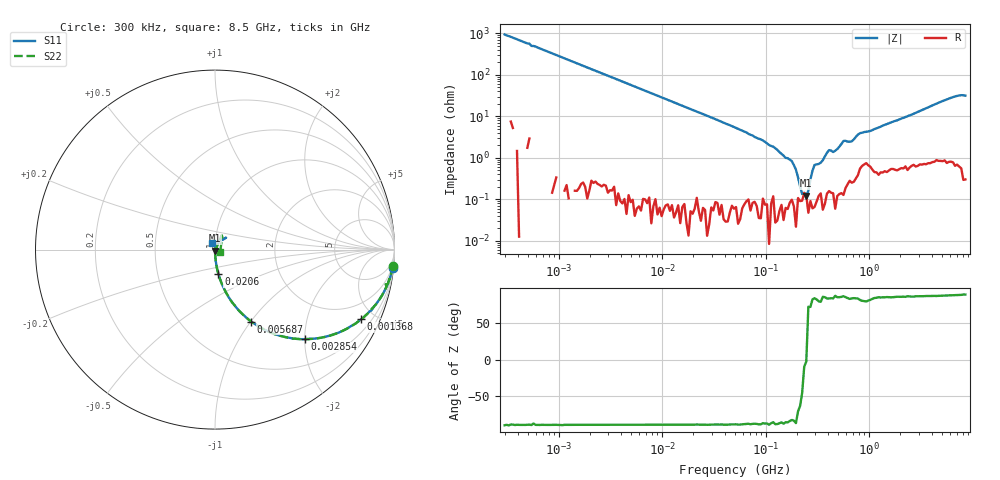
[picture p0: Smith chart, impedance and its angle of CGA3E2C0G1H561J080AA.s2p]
! S-parameter Generated by TDK Corporation
! Copyright(C) 2015 TDK Corporation.
! All Rights Reserved.
! TDK P/N: CGA3E2C0G1H561J080AA (Multilayer Ceramic Chip Capacitors)
! Property: C=560pF
! Size(LxWxT): 1.6x0.8x0.8mm, 0.063x0.031x0.031inches
! Model Type: s2p (Touchstone File Format Version 1.0)
! Frequency: DC=Yes Start=0.3MHz Stop=8500MHz 225points Log-sweep
! Note:
! Model Generated on Jun. 23, 2015
! Hash(MD5):
! Port Assignments:
!  1 ---| |--- 2
! Applicable Conditions:
!  Temperature = 25 degC
!  DC Bias Voltage = 0 V
!  Small Signal Operation
! Terms and conditions regarding TDK Simulation Models
! (1)This simulation model is being provided solely for informational purposes. Please refer to the specifications of the products in terms of detailed characteristics of such products.
! (2)In no event shall TDK Corporation of any of its subsidiaries be liable for any loss or damage arising, directly or indirectly,
!  From any information contained in this simulation model, including, but not limited to loss or damages arising from any inaccuracies, omissions or errors in connection with such information.
! (3)Any and all copyrights on this simulation model are owned by TDK Corporation.
!  Duplication or redistribution of this simulation model without prior written permission from TDK Corporation is prohibited.
! (4)This simulation model is subject to any modification or change without any prior notice.
! (5)Neither TDK Corporation nor any of its subsidiaries shall make any warranty, express or implied,
!  Including but not limited to the correctness, implied warranties of merchantability and fitness for a particular purpose with respect to this simulation models.
! (6)The use of this simulation model shall be deemed to have consented to the terms and conditions hereof.
# MHz S MA R 50
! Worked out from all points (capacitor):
!   224 points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, 300 kHz to 8.5 GHz, reference 50 ohm
!   read as one part in series: C = 558 pF near 314.1 kHz
!   lowest |Z| = 123 mohm at 246.6 MHz (marker M1)
!   series resonance near 247.1 MHz, so ESL is about 740 pH
!   S11 on the Smith chart (normalised r, x): 300 kHz: 1, -19; 1.368 MHz: 1.00, -4.19; 2.854 MHz: 1.00, -2.00; 5.687 MHz: 1.00, -1.00; 20.6 MHz: 1.00, -0.28; 8.5 GHz: 0.97, +0.07
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0.3  0.9944 -6.0  0.1053 84.8  0.1053 83.8  0.9944 -5.4
1.36767  0.902 -25.5  0.4316 64.5  0.4316 64.4  0.9019 -25.6
1.72111  0.856 -31.0  0.5164 58.9  0.5153 58.9  0.8558 -31.1
2.853835  0.7069 -44.9  0.7062 45.0  0.7061 45.0  0.707 -44.9
5.68736  0.4485 -63.4  0.8936 26.5  0.8935 26.6  0.4485 -63.4
9.430415  0.2898 -73.1  0.9568 16.8  0.9565 16.8  0.2896 -73.2
20.60362  0.1369 -82.0  0.9902 7.7  0.9895 7.7  0.1372 -82.1
51.67171  0.05416 -86.3  0.9982 2.9  0.9974 2.9  0.05412 -86.6
246.6485  0.006751 -78.1  0.9986 -0.4  0.9978 -0.3  0.005726 -91.7
283.1228  0.004162 -80.3  0.9992 -0.8  0.9994 -0.8  0.003521 -86.4
340.2802  0.002646 -58.2  0.9979 -1.0  0.9974 -0.9  0.0005997 -149.1
356.2888  0.001425 -36.5  0.9997 -1.0  0.9987 -1.0  0.0004958 163.4
373.0505  0.001041 -0.5  0.9989 -1.2  0.999 -1.2  0.001289 88.0
390.6008  0.001449 51.4  0.9983 -1.4  0.9975 -1.4  0.001721 74.3
564.2308  0.005646 65.7  0.9977 -2.6  0.999 -2.6  0.007632 89.2
618.5683  0.007476 63.7  0.9982 -2.4  0.9967 -2.5  0.006228 76.7
853.3868  0.01172 62.0  0.9927 -4.0  0.9936 -4.0  0.01264 51.7
1551.304  0.01332 71.7  0.994 -7.2  0.9941 -7.1  0.01394 58.5
2693.286  0.02088 65.6  0.9924 -12.3  0.9908 -12.2  0.02082 57.6
6450.987  0.08947 47.1  0.9855 -29.6  0.9866 -29.6  0.08762 65.3
7404.957  0.08567 47.9  0.9871 -33.9  0.9834 -33.8  0.08098 59.8
8500  0.03754 114.6  0.9892 -38.4  0.9901 -38.3  0.032 -24.4
